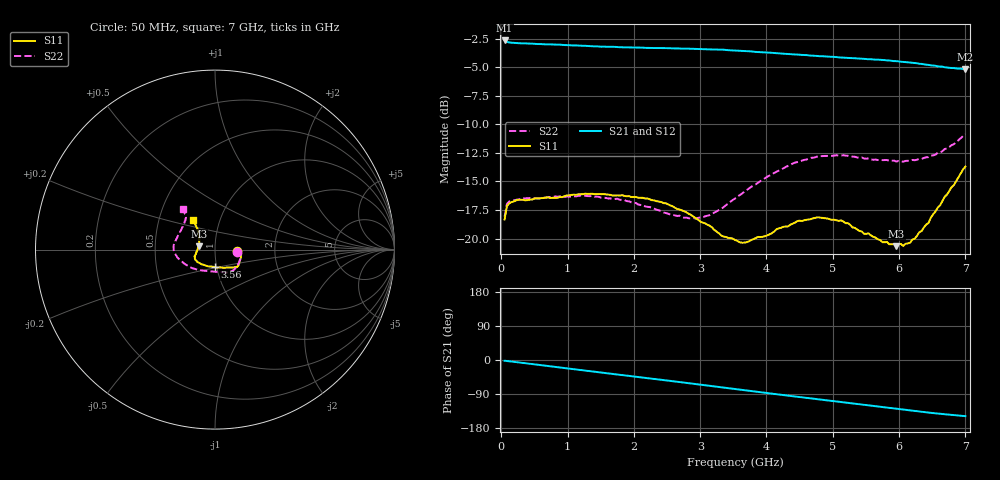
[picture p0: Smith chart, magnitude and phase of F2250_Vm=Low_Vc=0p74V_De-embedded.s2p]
! Integrated Device Technology
! Corporate Headquarters
! 6024 Silver Creek Valley Road
! San Jose, CA 95138  USA
! Phone:  1-408-284-8200
! Toll Free:  1-800-223-1366
! Webpage:  http://www.idt.com/
! Timing and RF Division
! 515 Groton Road, Suite 102
! Westford, MA 01886-6024
! Device:  F2250
! Description: Voltage Variable RF Attenuator
! Frequency:  50.0 -  6000.00 MHz
! Package:  3x3 mm Thin QFN Plastic Package: 16 pin
! Ports:  2 RF, 3 DC
!  Pin  1  = GND
!  Pin  2  = NC
!  Pin  3  = RF1  = Port 1
!  Pin  4  = NC
!  Pin  5  = GND
!  Pin  6  = GND
!  Pin  7  = GND
!  Pin  8  = GND
!  Pin  9  = NC
!  Pin 10  = RF2  = Port 2
!  Pin 11  = NC
!  Pin 12  = GND
!  Pin 13  = GND
!  Pin 14  = VCNTRL
!  Pin 15  = VDD
!  Pin 16  = VMODE
! Vcntrl:  0.740 Volts
! Vmode:  +0.000 Volts
! Vdd:  +3.30  Volts
! Current:  1.155 mA
! Data:  The device was measured on a the F2250 evaluation board which has
!  individual transmission lines to the RF pins.  Data was collected
!  using a calibrated network analyzer.  The evaluation board was
!  de-embedded using a TRL calibration technique.
!  The reference plane is the edge of the package pin.
! Misc:  SN 10
!  Action Tracker AT0258
! Date Measured:  2014-11-26
! Date:  2015-10-15  MJV
! Note:
!  Integrated Device Technology supplies this data as a sample of measured
!  data at the package pin for this product.  Your particular data for this
!  product may vary.
!  Data was taken at 25 degrees C.
!  Integrated Device Technology reserves the right to change this data at anytime.
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# GHz S dB R 50
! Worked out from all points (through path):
!   201 points, 50 MHz to 7 GHz, reference 50 ohm
!   highest |S21| = -2.66 dB at 50 MHz (marker M1); lowest = -5.2 dB at 7 GHz (marker M2)
!   group delay of S21, straight-line fit = 59.5 ps
!   lowest |S11| = -20.7 dB at 5.957 GHz (marker M3), VSWR 1.20, Z = 41.7 + j1.59 ohm
!   |S11| at or under -10 dB: start of sweep to end of sweep
!   |S22| runs from -18.2 to -10.9 dB; largest |S21 - S12| = 0.0018
!   S11 on the Smith chart (normalised r, x): 50 MHz: 1.28, -0.02; 3.56 GHz: 0.98, -0.19; 7 GHz: 0.74, +0.25
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0.05  -18.32 -4.3  -2.66 -2.0  -2.66 -2.0  -18.09 -5.7
0.08475  -17.16 -4.2  -2.78 -2.6  -2.80 -2.6  -16.96 -5.2
0.22375  -16.65 -7.5  -2.89 -5.6  -2.89 -5.5  -16.60 -9.9
0.745  -16.45 -22.0  -3.00 -16.9  -3.01 -16.9  -16.37 -29.5
1.2315  -16.11 -33.1  -3.13 -27.4  -3.12 -27.4  -16.26 -46.1
1.75275  -16.21 -39.4  -3.24 -38.3  -3.24 -38.3  -16.51 -57.9
2.37825  -16.76 -43.1  -3.32 -51.4  -3.32 -51.4  -17.52 -71.9
2.93425  -18.22 -54.2  -3.40 -63.5  -3.39 -63.5  -18.24 -96.7
3.14275  -18.87 -63.6  -3.45 -68.1  -3.44 -68.1  -17.94 -109.9
3.3165  -19.73 -74.1  -3.47 -72.0  -3.47 -72.0  -17.39 -120.3
3.525  -20.11 -88.4  -3.54 -76.6  -3.55 -76.6  -16.49 -132.0
3.55975  -20.20 -90.6  -3.56 -77.4  -3.55 -77.4  -16.34 -133.7
3.69875  -20.32 -102.2  -3.60 -80.5  -3.59 -80.5  -15.75 -140.6
4.1505  -19.19 -130.8  -3.78 -90.4  -3.76 -90.4  -14.14 -160.0
4.7065  -18.22 -151.7  -3.99 -102.3  -4.00 -102.3  -12.92 -175.5
5.1235  -18.39 -161.4  -4.15 -111.2  -4.15 -111.2  -12.73 174.8
5.85325  -20.50 174.1  -4.42 -126.5  -4.42 -126.5  -13.20 157.0
5.9575  -20.66 168.2  -4.47 -128.7  -4.47 -128.7  -13.25 154.1
6.166  -20.36 155.6  -4.59 -133.1  -4.59 -133.1  -13.19 147.4
6.444  -18.63 139.0  -4.80 -138.8  -4.80 -138.8  -12.87 138.1
6.722  -16.15 129.5  -5.02 -143.7  -5.02 -143.7  -12.11 131.0
7  -13.70 127.1  -5.18 -148.2  -5.18 -148.2  -10.86 128.5
